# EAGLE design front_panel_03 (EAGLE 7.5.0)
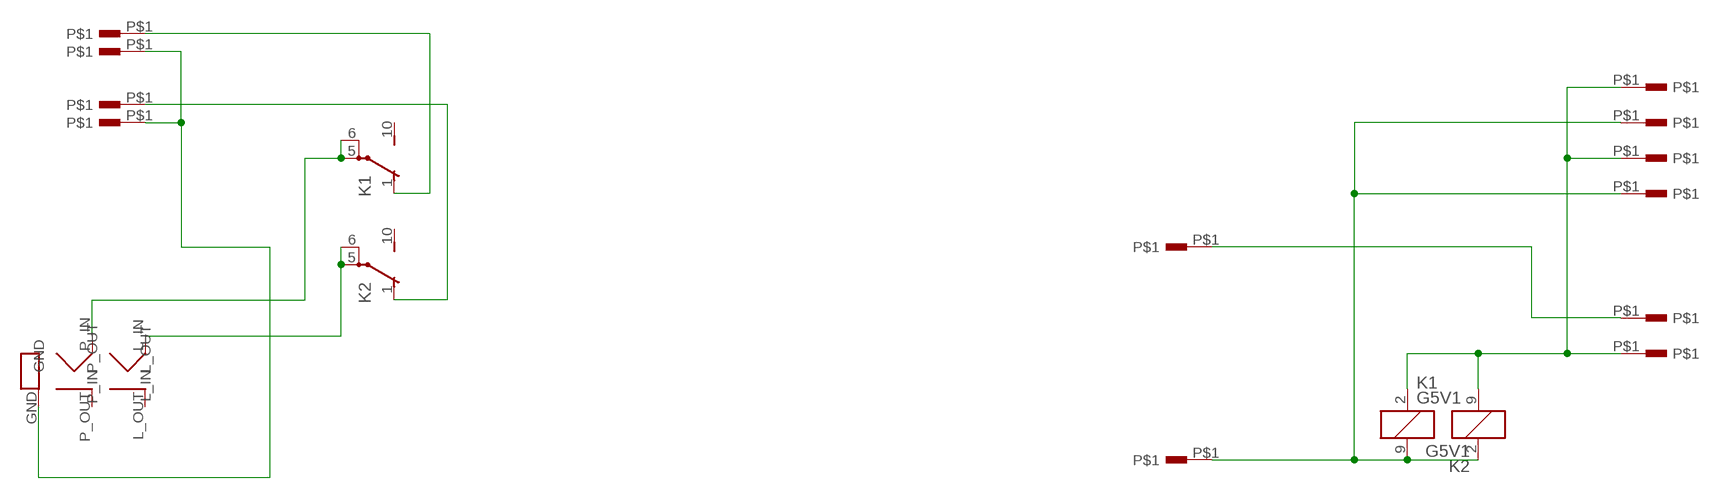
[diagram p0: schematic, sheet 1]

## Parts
K1  G5V1  [G5V1]
K2  G5V1  [G5V1]
U$1  ZAS6_3STS1  [ZAS6_3ST]
U$2  PIN  [PIN]
U$3  PIN  [PIN]
U$5  PIN  [PIN]
U$6  PIN  [PIN]
U$7  PIN  [PIN]
U$8  PIN  [PIN]
U$9  PIN  [PIN]
U$10  PIN  [PIN]
U$11  PIN  [PIN]
U$12  PIN  [PIN]
U$22  PIN  [PIN]
U$23  PIN  [PIN]

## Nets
GND2: U$1.GND U$22.P$1 U$23.P$1
N$1: K1.2 K2.9 U$6.P$1 U$8.P$1 U$10.P$1
N$3: U$3.P$1 U$5.P$1
N$5: K2.5(2:P) K2.6(2:P) U$1.L_IN
N$6: K1.5(2:P) K1.6(2:P) U$1.P_IN
N$7: K2.1(2:O) U$12.P$1
N$8: K1.1(2:O) U$11.P$1
N$16: K1.9 K2.2 U$2.P$1 U$7.P$1 U$9.P$1
Unconnected: K1.10(2:S) K2.10(2:S) U$1.L_OUT U$1.P_OUT

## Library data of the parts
K1 K2 = relay:G5V1: RELAY 1 x switch, 0.5 A/125 V AC, 1 A/24 V DC , Omron; MPN: G5V-1-DC24; OC_FARNELL: 9949593; OC_NEWARK: 36M6377
U$1 = lampy03:ZAS6_3ST
U$2 U$3 U$5-U$12 U$22 U$23 = lampy04:PIN

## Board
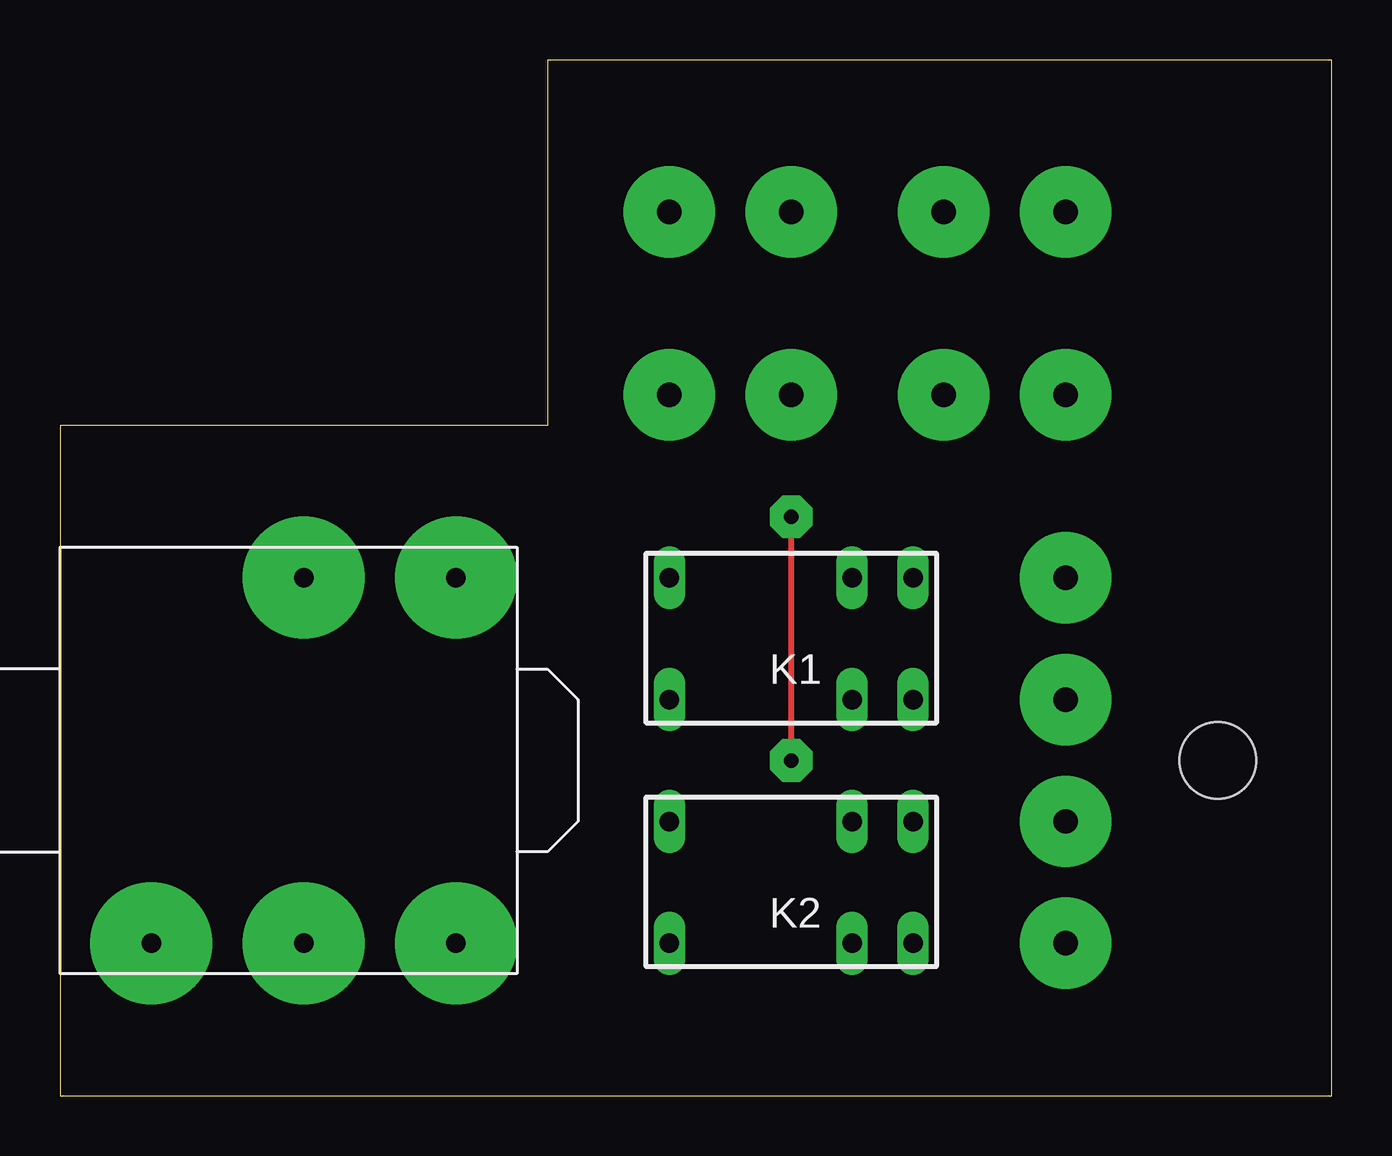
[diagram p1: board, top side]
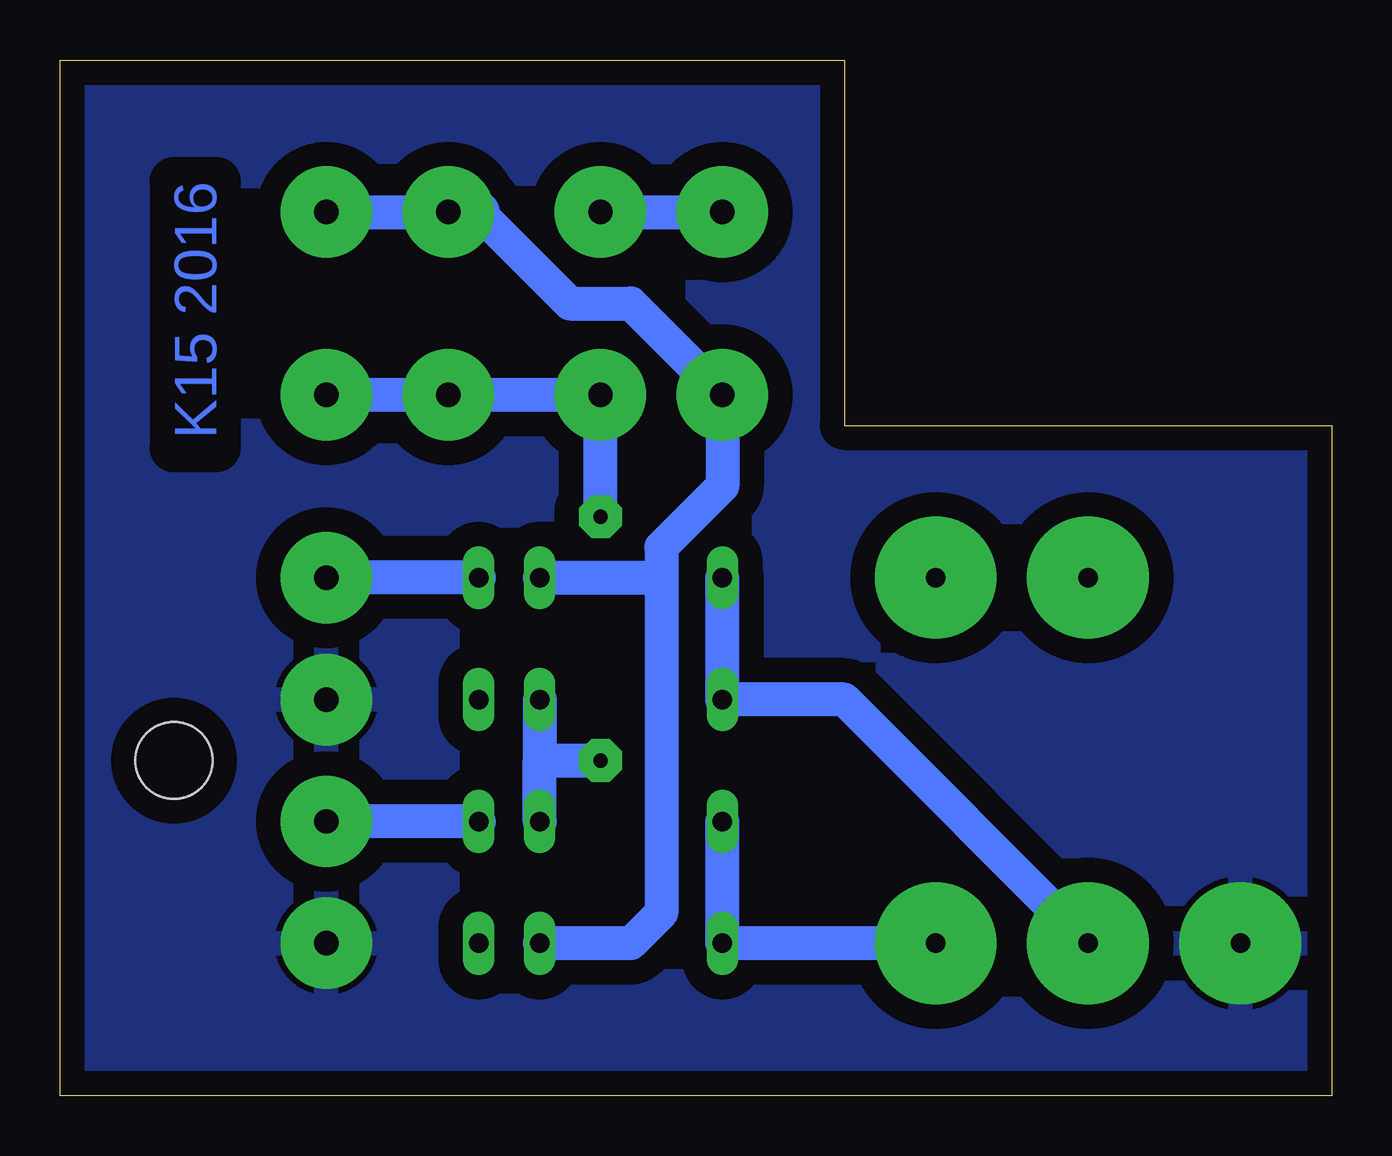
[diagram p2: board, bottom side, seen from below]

Size 53.01 x 43.17 mm. Coordinates in mm from the lower left corner, seen from the top.
Outline: 0,0 53.01,0 53.01,43.17 20.32,43.17 20.32,27.94 0,27.94 0,0
Copper layers (1*16): Top 0.035mm / dielectric 1.5mm / Bottom 0.035mm
Design rules "default": minimum track width 10mil, minimum drill 24mil, track to track 8mil, track to pad 8mil, pad to pad 8mil, via to via 8mil, smd to smd 8mil, copper to edge 40mil, drill to drill 8mil, minimum pad ring 10mil, minimum via ring 8mil, stop-mask expansion 4mil, vias tented up to drill 0mil, thermal gap 10mil
Holes 3.2 mm at 48.26,13.97

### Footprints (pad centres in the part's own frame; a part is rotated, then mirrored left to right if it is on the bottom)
G5V1 = drill 0.813 long: 1 -5.08,-2.54; 2 -2.54,-2.54; 5 5.08,-2.54; 6 5.08,2.54; 9 -2.54,2.54; 10 -5.08,2.54
ZAS6_3ST = drill 0.813 pad 5.08: GND -6.35,-7.62; L_IN 6.35,-7.62; L_OUT 6.35,7.62; P_IN 0,-7.62; P_OUT 0,7.62
PIN = drill 1.016 pad 3.81: P$1 0,0

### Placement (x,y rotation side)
K1  30.48,19.05 180 top
K2  30.48,8.89 180 top
U$1  10.16,13.97 0 top
U$2  36.83,29.21 0 top
U$3  25.4,36.83 0 top
U$5  30.48,36.83 0 top
U$6  36.83,36.83 0 top
U$7  41.91,29.21 0 top
U$8  25.4,29.21 0 top
U$9  30.48,29.21 0 top
U$10  41.91,36.83 0 top
U$11  41.91,21.59 0 top
U$12  41.91,11.43 0 top
U$22  41.91,6.35 0 top
U$23  41.91,16.51 0 top

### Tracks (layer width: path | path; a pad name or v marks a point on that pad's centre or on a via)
GND2
  pour Bottom (isolate 1.016): 0,0 0,43.18 54.61,43.18 54.61,0
N$1
  Bottom 1.422: 27.94,21.59 27.94,22.86 25.4,25.4 U$8.P$1 29.21,33.02 31.75,33.02 35.56,36.83 | 27.94,21.59 27.94,7.62 29.21,6.35 K2.9 | K1.2 27.94,21.59 | U$10.P$1 U$6.P$1
  Bottom 1.778: U$6.P$1 35.56,36.83
N$3
  Bottom 1.422: U$5.P$1 U$3.P$1
N$5
  Bottom 1.422: U$1.L_IN K2.6 K2.5
N$6
  Bottom 1.422: U$1.P_IN 20.32,16.51 K1.6 K1.5
N$7
  Bottom 1.422: K2.1 U$12.P$1
N$8
  Bottom 1.422: K1.1 U$11.P$1
N$16  (via drill 0.6 pad 1.78)
  Top 0.254: v30.48,13.97 v30.48,24.13
  Bottom 1.422: K2.2 33.02,13.97 | 33.02,13.97 v30.48,13.97 | K1.9 33.02,13.97 | v30.48,24.13 U$9.P$1 U$2.P$1 U$7.P$1

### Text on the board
Bottom: K15 2016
